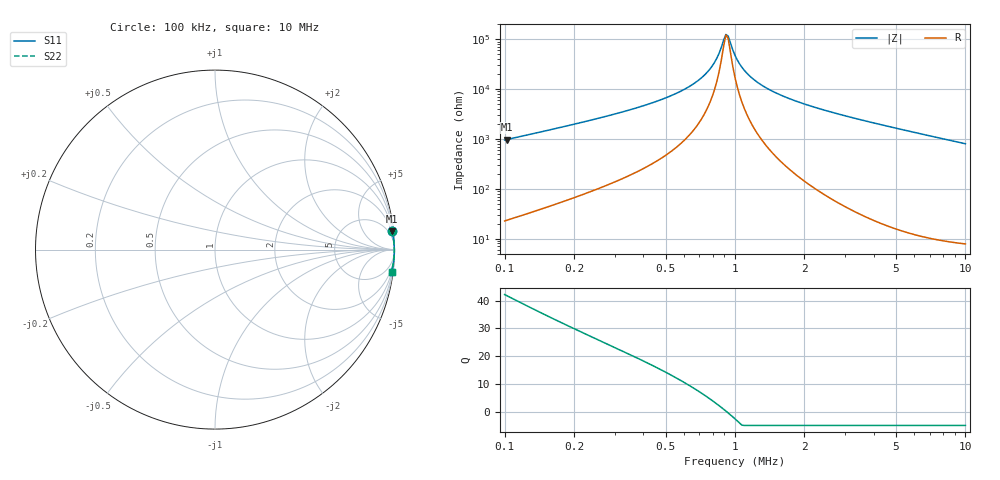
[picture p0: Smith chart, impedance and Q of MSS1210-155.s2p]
# MHz S MA R 50
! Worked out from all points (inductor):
!   203 points, 100 kHz to 10 MHz, reference 50 ohm
!   read as one part in series: L = 1.5 mH near 102.3 kHz
!   highest Q = 41.7 at 102.3 kHz (marker M1), where L = 1.52 mH
!   self-resonance near 912.8 kHz
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0.1  0.9921 6.0  0.104 -82.7  0.104 -82.7  0.9921 6.0
0.102306  0.9924 5.8  0.1017 -82.8  0.1017 -82.8  0.9924 5.8
0.1651284  0.9962 3.6  0.06197 -84.7  0.06197 -84.7  0.9962 3.6
0.2489084  0.9977 2.3  0.03944 -85.6  0.03944 -85.6  0.9977 2.3
0.6055893  0.999 0.6  0.00995 -83.9  0.00995 -83.9  0.999 0.6
0.7267518  0.9991 0.3  0.005534 -80.6  0.005534 -80.6  0.9991 0.3
0.7781962  0.9991 0.2  0.003946 -77.4  0.003946 -77.4  0.9991 0.2
0.8332822  0.9992 0.1  0.002406 -70.0  0.002406 -70.0  0.9992 0.1
0.9128429  0.9992 0.0  0.0007968 -11.2  0.0007968 -11.2  0.9992 0.0
0.9338928  0.9992 -0.0  0.0008576 25.6  0.0008576 25.6  0.9992 -0.0
1  0.9992 -0.1  0.00209 68.9  0.00209 68.9  0.9992 -0.1
1.046651  0.9993 -0.2  0.003098 76.2  0.003098 76.2  0.9993 -0.2
1.095479  0.9993 -0.2  0.004138 79.8  0.004138 79.8  0.9993 -0.2
1.173024  0.9993 -0.3  0.005731 82.7  0.005731 82.7  0.9993 -0.3
1.407715  0.9993 -0.6  0.01016 85.8  0.01016 85.8  0.9993 -0.6
1.768173  0.9993 -0.9  0.01622 87.0  0.01622 87.0  0.9993 -0.9
2.43298  0.9991 -1.5  0.02619 87.3  0.02619 87.3  0.9991 -1.5
3.424944  0.9987 -2.3  0.03989 87.0  0.03989 87.0  0.9987 -2.3
5.162633  0.9975 -3.6  0.06266 85.9  0.06266 85.9  0.9975 -3.6
6.787083  0.9958 -4.8  0.08337 84.7  0.08337 84.7  0.9958 -4.8
8.524974  0.9935 -6.0  0.1052 83.4  0.1052 83.4  0.9935 -6.0
10  0.9911 -7.1  0.1235 82.3  0.1235 82.3  0.9911 -7.1
